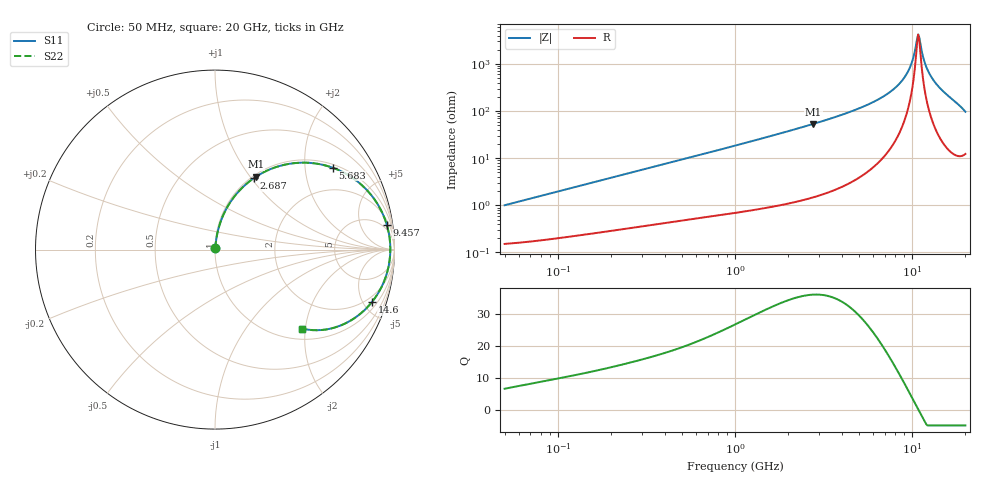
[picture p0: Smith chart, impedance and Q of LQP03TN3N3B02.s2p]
!Murata Part Number: LQP03TN3N3B02
!These Parameters are Measured in Series Mode Connection
!  o--[Z]--o
!Port1  Port2
!  o-------o
!Freq. Start=50[MHz] Stop=20[GHz], 401[Steps]
# Hz S RI R 50
!Freq.(Hz) S11(Real) S11(Imag) S21(Real) S21(Imag) S12(Real) S12(Imag) S22(Real) S22(Imag)
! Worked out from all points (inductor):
!   401 points, 50 MHz to 20 GHz, reference 50 ohm
!   read as one part in series: L = 3.15 nH near 51.52 MHz
!   highest Q = 36.1 at 2.769 GHz (marker M1), where L = 3.07 nH
!   self-resonance near 10.82 GHz
!   S11 on the Smith chart (normalised r, x): 50 MHz: 1.00, +0.02; 2.687 GHz: 1.03, +1.03; 5.683 GHz: 1.11, +2.79; 9.457 GHz: 3, +13; 14.6 GHz: 1.48, -5.75; 20 GHz: 1.25, -1.92
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5e7  0.00162 0.00991  0.9984 -0.00991  0.9984 -0.00991  0.00162 0.00991
1.364002e8  0.00303 0.0262  0.997 -0.0262  0.997 -0.0262  0.00303 0.0262
3.721004e8  0.00881 0.0688  0.9912 -0.0688  0.9912 -0.0688  0.00881 0.0688
1e9  0.0391 0.1759  0.9609 -0.1759  0.9609 -0.1759  0.0391 0.1759
1.740566e9  0.102 0.288  0.898 -0.288  0.898 -0.288  0.102 0.288
2.687447e9  0.2169 0.3985  0.7831 -0.3985  0.7831 -0.3985  0.2169 0.3985
2.728004e9  0.2224 0.4023  0.7776 -0.4023  0.7776 -0.4023  0.2224 0.4023
2.769174e9  0.2281 0.406  0.7719 -0.406  0.7719 -0.406  0.2281 0.406
4.212059e9  0.4431 0.4819  0.5569 -0.4819  0.5569 -0.4819  0.4431 0.4819
5.683258e9  0.655 0.4566  0.345 -0.4566  0.345 -0.4566  0.655 0.4566
7.442007e9  0.8455 0.3324  0.1545 -0.3324  0.1545 -0.3324  0.8455 0.3324
8.516016e9  0.919 0.2307  0.081 -0.2307  0.081 -0.2307  0.919 0.2307
9.457416e9  0.9577 0.1364  0.0423 -0.1364  0.0423 -0.1364  0.9577 0.1364
9.892087e9  0.9682 0.0929  0.0318 -0.0929  0.0318 -0.0929  0.9682 0.0929
1.050288e10  0.9759 0.0329  0.0241 -0.0329  0.0241 -0.0329  0.9759 0.0329
1.082228e10  0.9769 0.00228  0.0231 -0.00228  0.0231 -0.00228  0.9769 0.00228
1.115139e10  0.976 -0.0285  0.024 0.0285  0.024 0.0285  0.976 -0.0285
1.166392e10  0.9707 -0.0748  0.0293 0.0748  0.0293 0.0748  0.9707 -0.0748
1.238412e10  0.9565 -0.1361  0.0435 0.1361  0.0435 0.1361  0.9565 -0.1361
1.460232e10  0.8735 -0.2932  0.1265 0.2932  0.1265 0.2932  0.8735 -0.2932
1.747767e10  0.7022 -0.4218  0.2978 0.4218  0.2978 0.4218  0.7022 -0.4218
2e10  0.4845 -0.4396  0.5155 0.4396  0.5155 0.4396  0.4845 -0.4396
